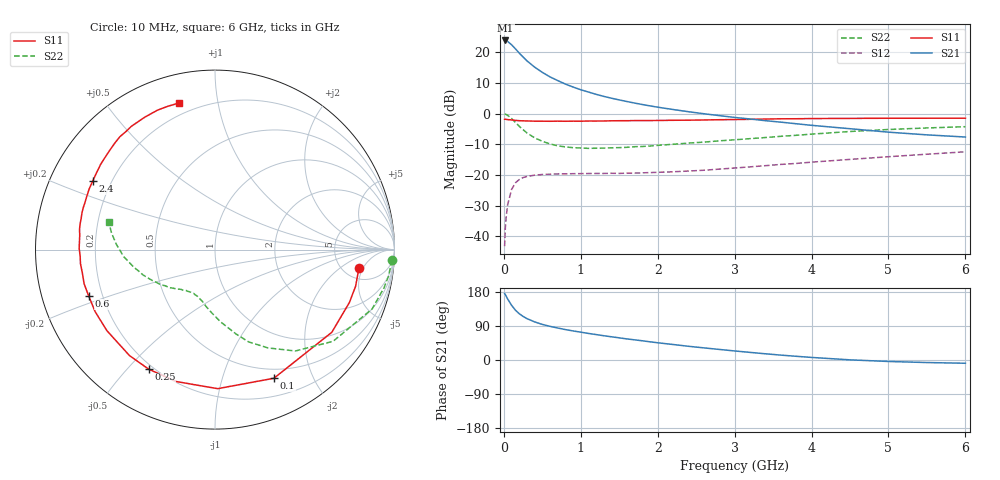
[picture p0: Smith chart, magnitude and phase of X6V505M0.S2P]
! SIEMENS Small Signal Semiconductors
! BFP193W
! Si NPN RF Bipolar Junction Transistor in SOT343
! VCE = 0.5 V  IC = 5 mA
! Common Emitter S-Parameters:  April 1994
# GHz  S  MA  R  50
!  f  S11  S21  S12  S22
! GHz  MAG  ANG  MAG  ANG  MAG  ANG  MAG  ANG
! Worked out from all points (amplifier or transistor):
!   40 points, 10 MHz to 6 GHz, reference 50 ohm
!   highest |S21| = 23.8 dB at 20 MHz (marker M1)
!   |S21| within 3 dB of that: start of sweep to 160.3 MHz
!   unconditionally stable (mu >= 1): 1.527 GHz to end of sweep
!   at 200 MHz: K = 0.15, MSG = 20.6 dB, |S12| = -21.5 dB
!   at 1.5 GHz: K = 0.99, MSG = 12.0 dB, |S12| = -19.5 dB
!   at 6 GHz: K = 1.14, MAG = 0.1 dB, |S12| = -12.5 dB
!   S11 on the Smith chart (normalised r, x): 10 MHz: 7.01, -4.11; 100 MHz: 0.39, -1.49; 250 MHz: 0.18, -0.57; 600 MHz: 0.15, -0.17; 2.4 GHz: 0.13, +0.26; 6 GHz: 0.14, +0.77
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0.01  0.8087 -7.2  15.55 175.3  0.0069 86.9  0.9868 -3.4
0.02  0.8096 -14.6  15.57 172.2  0.0141 82.2  0.9782 -8.7
0.03  0.8047 -21.5  15.41 168.4  0.0205 79.7  0.9655 -12.7
0.05  0.7974 -35.3  14.98 160.9  0.0328 72.5  0.9357 -20.7
0.1  0.7884 -65.4  13.27 144.6  0.0576 57.5  0.8332 -37.8
0.15  0.775 -88.9  11.4 131.6  0.0743 46.5  0.7208 -51.6
0.2  0.766 -106.3  9.695 122.2  0.084 38.8  0.6221 -61.7
0.25  0.7618 -119.0  8.36 115.0  0.0906 32.9  0.5471 -70.0
0.3  0.7587 -128.9  7.252 109.3  0.0944 29.1  0.4845 -76.0
0.4  0.7528 -143.1  5.725 100.6  0.0991 23.7  0.4028 -85.7
0.5  0.752 -152.6  4.699 93.9  0.1017 20.5  0.3533 -92.9
0.6  0.7497 -159.8  3.967 88.8  0.1028 18.4  0.3208 -98.9
0.8  0.7503 -170.0  3.029 80.3  0.1043 16.3  0.2865 -107.2
1.1  0.7568 179.6  2.246 70.1  0.1055 15.7  0.2712 -116.2
1.3  0.7578 174.0  1.907 64.0  0.1057 16.3  0.2739 -120.7
1.6  0.7658 166.6  1.574 55.6  0.107 18.2  0.2821 -126.4
2.2  0.7781 154.4  1.166 40.9  0.1126 23.1  0.316 -137.0
2.4  0.7813 150.6  1.073 36.2  0.1157 24.8  0.3306 -140.2
3.2  0.8065 136.5  0.817 20.1  0.1354 30.2  0.3905 -154.0
4.5  0.8352 117.9  0.567 0.4  0.1792 31.2  0.5109 -175.7
5.5  0.8407 108.3  0.45 -6.7  0.2176 28.4  0.5835 170.9
6  0.8409 103.8  0.415 -8.6  0.2384 26.5  0.6119 165.5
